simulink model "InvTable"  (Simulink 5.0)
settings: Solver=FixedStepDiscrete  StartTime=0.0  StopTime=inf  FixedStep=samplePeriod  RelTol=1e-3
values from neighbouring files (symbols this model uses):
  a0 = zeros(1, nAct)    [initialize.m]    (also in quake.m = 0; rspect.m = 1)
  azMask = zeros(nAcc, 1)    [initialize.m]
  bal = [[ 1  1  1  1  0  0  0  0  0  0  0  0]    [initialize.m]
  cmap = jet    [initialize.m]    (also in tableAnimation.m = self.cmap)
  ea_t = zeros(3, nAcc)    [initialize.m]
  faces = nAct               			+ [ 1  2  3  4    [initialize.m]    (also in tableAnimation.m = self.faces)
  flowCanon = 63090.2    [initialize.m]
  fmax = zeros(nAct, 1)    [initialize.m]
  gasConstant = 1.8    [initialize.m]
  gee = 1.0    (= 1)    [initialize.m]    (also in accelA2T.m = h(24); accelT2A.m = h(24); Test.m)
  iactParamsX = [actParamsX, dfGain, solver]    [initialize.m]
  iactParamsY = [actParamsY, dfGain, solver]    [initialize.m]
  iactParamsZ = [actParamsZ, dfGain, solver]    [initialize.m]
  inertia = [Ixx 0 0; 0 Iyy 0; 0 0 Izz]    [initialize.m]
  inertiaCanon = 0.1130    (= 0.113)    [initialize.m]
  linAccelCanon = 9800.0    (= 9800)    [initialize.m]    (also in accelA2T.m = h(19); accelT2A.m = h(19); Test.m)
  lines = nAct               			+ [ 1  2  3  4  1    				5  6  7  8  5    				9 10 11 12  9    				0  2  6 10       				0  3  7 11       				0  4  8 12  0];  	lines(find(lines==nAct)) = 0    [initialize.m]    (also in tableAnimation.m = self.lines; viewer.m = 1)
  linVelocCanon = 1000.0    (= 1000)    [initialize.m]    (also in Test.m)
  mass = [massX massY massZ]'    [initialize.m]
  massCanon = 0.4535924e-06    (= 4.535924e-07)    [initialize.m]
  maxDispl = [maxDisplX  			maxDisplY  			maxDisplZ  			maxDisplZ * linVelocCanon / rollRadius  * 180/pi  			maxDisplZ * linVelocCanon / pitchRadius * 180/pi  			min(maxDisplX, maxDisplY) * linVelocCanon / yawRadius * 180/pi]    [initialize.m]
  maxOilVolume = volume * (1 - (precharge/supplyPress)^(1/gasConstant))    (= 32.2704137442)    [initialize.m]
  maxVeloc = [maxVelocX  			maxVelocY  			maxVelocZ  			maxVelocZ * linVelocCanon / rollRadius  * 180/pi  			maxVelocZ * linVelocCanon / pitchRadius * 180/pi  			min(maxVelocX, maxVelocY) * linVelocCanon / yawRadius * 180/pi]    [initialize.m]
  minDispl = -maxDispl    [initialize.m]
  minVeloc = -maxVeloc    [initialize.m]
  nAct = size(rt_t, 2)    [initialize.m]    (also in tableAnimation.m = self.nAct)
  precharge = 2000    [initialize.m]
  pumpFlow = 1e10    (= 10000000000)    [initialize.m]
  ra_t = [  -20.0   -20.0   -92.0 -2590.0  2590.0   -62.0 -2133.0 -2133.0  2133.0  2133.0   -62.0    [initialize.m]    (also in accelA2T.m = [-h9   -h9 -h15 -h10  h10 -h14 -h12 -h12  h12  h12 -h16; accelT2A.m = [-h9   -h9 -h15 -h10  h10 -h14 -h12 -h12  h12  h12 -h16)
  rb_w = [-5692.1 -5692.1  5692.1  5692.1 -2500.0 -2500.0  2500.0  2500.0 -2400.0 -2400.0  2400.0  2400.0    [initialize.m]    (also in tableAnimation.m = rtxrb_w(:,end-nAct+1:end); positT2A.m = [-h4 -h4  h4  h4 -h1 -h1  h1  h1 -h6 -h6  h6  h6)
  returnPress = 50    [initialize.m]
  rgt = -rtg    [initialize.m]
  roll = tbl(4)    [positT2A.m]
  rotAccelCanon = 1    [initialize.m]    (also in accelA2T.m = h(22); accelT2A.m = h(22); Test.m)
  rotForceCanon = 1000    [initialize.m]    (also in forceA2T.m = h(23); Test.m)
  rotVelocCanon = 1    [initialize.m]    (also in accelA2T.m = h(21); accelT2A.m = h(21); Test.m)
  rt_t = [-3106.4 -3106.4  3106.4  3106.4 -2500.0 -2500.0  2500.0  2500.0 -2400.0 -2400.0  2400.0  2400.0    [initialize.m]    (also in positT2A.m = [rt_tx rt_ty rt_tz])
  rtg = cg    [initialize.m]
  rtx_t = [rt_t	topPlane.topLeft(:)  topPlane.topRight(:)  					topPlane.botRight(:) topPlane.botLeft(:)   					midPlane.topLeft(:)  midPlane.topRight(:)  					midPlane.botRight(:) midPlane.botLeft(:)   					botPlane.topLeft(:)  botPlane.topRight(:)  					botPlane.botRight(:) botPlane.botLeft(:)]    [initialize.m]
  samplePeriod = 1/1024    (= 0.0009765625)    [initialize.m]    (also in viewer.m = eval(getHeaderValue(header, 'DELTA_T')))
  supplyPress = 3000    [initialize.m]
  volume = 160    [initialize.m]    (also in quake.m = volume / 231.0)
  volumeCanon = 3785412.0    (= 3785412)    [initialize.m]
  zlim = [min(rb_w(3,:)) 2*halfLengthZ*lengthCanon]    [initialize.m]
undefined symbols (not defined in the file or in its folder): magnitude
libraries: aerospace x51, simulink x26, simulink_extras x1
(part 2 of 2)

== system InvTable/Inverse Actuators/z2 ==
  note: Parameter vector: 1: oil bulk modulus (force/displ^2) 2: servovalve natural frequency (Hz) 3: servovalve damping ratio 4: servovalve overlap 5: rated pressure (force/displ^2) 6: flow at rated pressure (displ^3/sec) 7: actuator piston area 1 (displ^2) 8: actuator piston area 2 (displ^2) 9: actuator usable stroke 1 (displ) 10: actuator usable stroke 2 (displ) 11: actuator end cushion length 1 (displ) 12: actuator end cushion length 2 (displ) 13: actuator parasitic damping factor 14: cross-chamber leakage factor (flow/press) 15: ratio port openings according to area 16: sample period (sec) Conversion factors used for converting signals from external (user) to internal (canonical) units: 17: displacement 18: velocity 19: force 20: pressure 21: flow Other: 22: delta-F feedback gain 23: inverse solver (0: exact, 1: approx)
  note: Note: "1" and "2" denote actuator cylinders on either side of the actuator piston. With positive valve drive, oil is ported into cylinder 1, resulting in positive displacement.
  note: Auxiliary diagnostic output vector: 1: valve opening 2: C1 pressure 3: C2 pressure 4: delta pressure 5: force 6: velocity 7: C1 flow 8: C2 flow 9: total flow 10: kinematic flow 11: compressibility flow 12: leakage flow 13: iteration error
  displ : Inport
  veloc : Inport  Port=2
  force : Inport  Port=3
  spl press : Inport  Port=4
  rtn press : Inport  Port=5
  abs : Abs
  invactuator : S-Function  FunctionName=invactuator  Parameters=params
  total flow sel : Selector  Elements=9  InputPortWidth=13
  cmd : Outport
  flow : Outport  Port=2
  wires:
  abs/1 -> flow/1
  total flow sel/1 -> abs/1
  invactuator/2 -> total flow sel/1
  force/1 -> invactuator/3
  veloc/1 -> invactuator/2
  invactuator/1 -> cmd/1
  displ/1 -> invactuator/1
  rtn press/1 -> invactuator/5
  spl press/1 -> invactuator/4

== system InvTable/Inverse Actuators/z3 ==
  note: Auxiliary diagnostic output vector: 1: valve opening 2: C1 pressure 3: C2 pressure 4: delta pressure 5: force 6: velocity 7: C1 flow 8: C2 flow 9: total flow 10: kinematic flow 11: compressibility flow 12: leakage flow 13: iteration error
  note: Note: "1" and "2" denote actuator cylinders on either side of the actuator piston. With positive valve drive, oil is ported into cylinder 1, resulting in positive displacement.
  note: Parameter vector: 1: oil bulk modulus (force/displ^2) 2: servovalve natural frequency (Hz) 3: servovalve damping ratio 4: servovalve overlap 5: rated pressure (force/displ^2) 6: flow at rated pressure (displ^3/sec) 7: actuator piston area 1 (displ^2) 8: actuator piston area 2 (displ^2) 9: actuator usable stroke 1 (displ) 10: actuator usable stroke 2 (displ) 11: actuator end cushion length 1 (displ) 12: actuator end cushion length 2 (displ) 13: actuator parasitic damping factor 14: cross-chamber leakage factor (flow/press) 15: ratio port openings according to area 16: sample period (sec) Conversion factors used for converting signals from external (user) to internal (canonical) units: 17: displacement 18: velocity 19: force 20: pressure 21: flow Other: 22: delta-F feedback gain 23: inverse solver (0: exact, 1: approx)
  displ : Inport
  veloc : Inport  Port=2
  force : Inport  Port=3
  spl press : Inport  Port=4
  rtn press : Inport  Port=5
  abs : Abs
  invactuator : S-Function  FunctionName=invactuator  Parameters=params
  total flow sel : Selector  Elements=9  InputPortWidth=13
  cmd : Outport
  flow : Outport  Port=2
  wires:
  spl press/1 -> invactuator/4
  rtn press/1 -> invactuator/5
  displ/1 -> invactuator/1
  invactuator/1 -> cmd/1
  veloc/1 -> invactuator/2
  force/1 -> invactuator/3
  invactuator/2 -> total flow sel/1
  total flow sel/1 -> abs/1
  abs/1 -> flow/1

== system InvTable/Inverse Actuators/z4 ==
  note: Parameter vector: 1: oil bulk modulus (force/displ^2) 2: servovalve natural frequency (Hz) 3: servovalve damping ratio 4: servovalve overlap 5: rated pressure (force/displ^2) 6: flow at rated pressure (displ^3/sec) 7: actuator piston area 1 (displ^2) 8: actuator piston area 2 (displ^2) 9: actuator usable stroke 1 (displ) 10: actuator usable stroke 2 (displ) 11: actuator end cushion length 1 (displ) 12: actuator end cushion length 2 (displ) 13: actuator parasitic damping factor 14: cross-chamber leakage factor (flow/press) 15: ratio port openings according to area 16: sample period (sec) Conversion factors used for converting signals from external (user) to internal (canonical) units: 17: displacement 18: velocity 19: force 20: pressure 21: flow Other: 22: delta-F feedback gain 23: inverse solver (0: exact, 1: approx)
  note: Note: "1" and "2" denote actuator cylinders on either side of the actuator piston. With positive valve drive, oil is ported into cylinder 1, resulting in positive displacement.
  note: Auxiliary diagnostic output vector: 1: valve opening 2: C1 pressure 3: C2 pressure 4: delta pressure 5: force 6: velocity 7: C1 flow 8: C2 flow 9: total flow 10: kinematic flow 11: compressibility flow 12: leakage flow 13: iteration error
  displ : Inport
  veloc : Inport  Port=2
  force : Inport  Port=3
  spl press : Inport  Port=4
  rtn press : Inport  Port=5
  abs : Abs
  invactuator : S-Function  FunctionName=invactuator  Parameters=params
  total flow sel : Selector  Elements=9  InputPortWidth=13
  cmd : Outport
  flow : Outport  Port=2
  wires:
  abs/1 -> flow/1
  total flow sel/1 -> abs/1
  invactuator/2 -> total flow sel/1
  force/1 -> invactuator/3
  veloc/1 -> invactuator/2
  invactuator/1 -> cmd/1
  displ/1 -> invactuator/1
  rtn press/1 -> invactuator/5
  spl press/1 -> invactuator/4

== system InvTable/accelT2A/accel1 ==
  linacc : Inport
  rotacc : Inport  Port=2
  rotvel : Inport  Port=3
  Sum : Sum  Inputs=+++
  crossprod1 : aerospace/Axes Transformations/3x3 cross product
  crossprod2 : aerospace/Axes Transformations/3x3 cross product
  crossprod3 : aerospace/Axes Transformations/3x3 cross product
  dotprod : simulink/Math Operations/Dot Product
  orient : Constant  Value=ea_t(:,id)
  ra_t : Constant  Value=ra_t(:,id)
  out : Outport
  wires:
  crossprod2/1 -> crossprod3/2
  crossprod3/1 -> Sum/3
  rotvel/1 -> crossprod3/1, crossprod2/1
  crossprod1/1 -> Sum/2
  ra_t/1 -> crossprod2/2, crossprod1/2
  rotacc/1 -> crossprod1/1
  Sum/1 -> dotprod/1
  linacc/1 -> Sum/1
  dotprod/1 -> out/1
  orient/1 -> dotprod/2

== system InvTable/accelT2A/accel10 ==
  linacc : Inport
  rotacc : Inport  Port=2
  rotvel : Inport  Port=3
  Sum : Sum  Inputs=+++
  crossprod1 : aerospace/Axes Transformations/3x3 cross product
  crossprod2 : aerospace/Axes Transformations/3x3 cross product
  crossprod3 : aerospace/Axes Transformations/3x3 cross product
  dotprod : simulink/Math Operations/Dot Product
  orient : Constant  Value=ea_t(:,id)
  ra_t : Constant  Value=ra_t(:,id)
  out : Outport
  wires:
  orient/1 -> dotprod/2
  dotprod/1 -> out/1
  linacc/1 -> Sum/1
  Sum/1 -> dotprod/1
  rotacc/1 -> crossprod1/1
  ra_t/1 -> crossprod1/2, crossprod2/2
  crossprod1/1 -> Sum/2
  rotvel/1 -> crossprod2/1, crossprod3/1
  crossprod3/1 -> Sum/3
  crossprod2/1 -> crossprod3/2

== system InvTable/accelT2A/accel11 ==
  linacc : Inport
  rotacc : Inport  Port=2
  rotvel : Inport  Port=3
  Sum : Sum  Inputs=+++
  crossprod1 : aerospace/Axes Transformations/3x3 cross product
  crossprod2 : aerospace/Axes Transformations/3x3 cross product
  crossprod3 : aerospace/Axes Transformations/3x3 cross product
  dotprod : simulink/Math Operations/Dot Product
  orient : Constant  Value=ea_t(:,id)
  ra_t : Constant  Value=ra_t(:,id)
  out : Outport
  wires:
  crossprod2/1 -> crossprod3/2
  crossprod3/1 -> Sum/3
  rotvel/1 -> crossprod3/1, crossprod2/1
  crossprod1/1 -> Sum/2
  ra_t/1 -> crossprod2/2, crossprod1/2
  rotacc/1 -> crossprod1/1
  Sum/1 -> dotprod/1
  linacc/1 -> Sum/1
  dotprod/1 -> out/1
  orient/1 -> dotprod/2

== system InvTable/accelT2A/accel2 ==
  linacc : Inport
  rotacc : Inport  Port=2
  rotvel : Inport  Port=3
  Sum : Sum  Inputs=+++
  crossprod1 : aerospace/Axes Transformations/3x3 cross product
  crossprod2 : aerospace/Axes Transformations/3x3 cross product
  crossprod3 : aerospace/Axes Transformations/3x3 cross product
  dotprod : simulink/Math Operations/Dot Product
  orient : Constant  Value=ea_t(:,id)
  ra_t : Constant  Value=ra_t(:,id)
  out : Outport
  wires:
  orient/1 -> dotprod/2
  dotprod/1 -> out/1
  linacc/1 -> Sum/1
  Sum/1 -> dotprod/1
  rotacc/1 -> crossprod1/1
  ra_t/1 -> crossprod1/2, crossprod2/2
  crossprod1/1 -> Sum/2
  rotvel/1 -> crossprod2/1, crossprod3/1
  crossprod3/1 -> Sum/3
  crossprod2/1 -> crossprod3/2

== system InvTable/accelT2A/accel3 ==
  linacc : Inport
  rotacc : Inport  Port=2
  rotvel : Inport  Port=3
  Sum : Sum  Inputs=+++
  crossprod1 : aerospace/Axes Transformations/3x3 cross product
  crossprod2 : aerospace/Axes Transformations/3x3 cross product
  crossprod3 : aerospace/Axes Transformations/3x3 cross product
  dotprod : simulink/Math Operations/Dot Product
  orient : Constant  Value=ea_t(:,id)
  ra_t : Constant  Value=ra_t(:,id)
  out : Outport
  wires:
  crossprod2/1 -> crossprod3/2
  crossprod3/1 -> Sum/3
  rotvel/1 -> crossprod3/1, crossprod2/1
  crossprod1/1 -> Sum/2
  ra_t/1 -> crossprod2/2, crossprod1/2
  rotacc/1 -> crossprod1/1
  Sum/1 -> dotprod/1
  linacc/1 -> Sum/1
  dotprod/1 -> out/1
  orient/1 -> dotprod/2

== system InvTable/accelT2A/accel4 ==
  linacc : Inport
  rotacc : Inport  Port=2
  rotvel : Inport  Port=3
  Sum : Sum  Inputs=+++
  crossprod1 : aerospace/Axes Transformations/3x3 cross product
  crossprod2 : aerospace/Axes Transformations/3x3 cross product
  crossprod3 : aerospace/Axes Transformations/3x3 cross product
  dotprod : simulink/Math Operations/Dot Product
  orient : Constant  Value=ea_t(:,id)
  ra_t : Constant  Value=ra_t(:,id)
  out : Outport
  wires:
  orient/1 -> dotprod/2
  dotprod/1 -> out/1
  linacc/1 -> Sum/1
  Sum/1 -> dotprod/1
  rotacc/1 -> crossprod1/1
  ra_t/1 -> crossprod1/2, crossprod2/2
  crossprod1/1 -> Sum/2
  rotvel/1 -> crossprod2/1, crossprod3/1
  crossprod3/1 -> Sum/3
  crossprod2/1 -> crossprod3/2

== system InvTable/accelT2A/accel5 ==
  linacc : Inport
  rotacc : Inport  Port=2
  rotvel : Inport  Port=3
  Sum : Sum  Inputs=+++
  crossprod1 : aerospace/Axes Transformations/3x3 cross product
  crossprod2 : aerospace/Axes Transformations/3x3 cross product
  crossprod3 : aerospace/Axes Transformations/3x3 cross product
  dotprod : simulink/Math Operations/Dot Product
  orient : Constant  Value=ea_t(:,id)
  ra_t : Constant  Value=ra_t(:,id)
  out : Outport
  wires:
  crossprod2/1 -> crossprod3/2
  crossprod3/1 -> Sum/3
  rotvel/1 -> crossprod3/1, crossprod2/1
  crossprod1/1 -> Sum/2
  ra_t/1 -> crossprod2/2, crossprod1/2
  rotacc/1 -> crossprod1/1
  Sum/1 -> dotprod/1
  linacc/1 -> Sum/1
  dotprod/1 -> out/1
  orient/1 -> dotprod/2

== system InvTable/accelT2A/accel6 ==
  linacc : Inport
  rotacc : Inport  Port=2
  rotvel : Inport  Port=3
  Sum : Sum  Inputs=+++
  crossprod1 : aerospace/Axes Transformations/3x3 cross product
  crossprod2 : aerospace/Axes Transformations/3x3 cross product
  crossprod3 : aerospace/Axes Transformations/3x3 cross product
  dotprod : simulink/Math Operations/Dot Product
  orient : Constant  Value=ea_t(:,id)
  ra_t : Constant  Value=ra_t(:,id)
  out : Outport
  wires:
  orient/1 -> dotprod/2
  dotprod/1 -> out/1
  linacc/1 -> Sum/1
  Sum/1 -> dotprod/1
  rotacc/1 -> crossprod1/1
  ra_t/1 -> crossprod1/2, crossprod2/2
  crossprod1/1 -> Sum/2
  rotvel/1 -> crossprod2/1, crossprod3/1
  crossprod3/1 -> Sum/3
  crossprod2/1 -> crossprod3/2

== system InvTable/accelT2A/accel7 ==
  linacc : Inport
  rotacc : Inport  Port=2
  rotvel : Inport  Port=3
  Sum : Sum  Inputs=+++
  crossprod1 : aerospace/Axes Transformations/3x3 cross product
  crossprod2 : aerospace/Axes Transformations/3x3 cross product
  crossprod3 : aerospace/Axes Transformations/3x3 cross product
  dotprod : simulink/Math Operations/Dot Product
  orient : Constant  Value=ea_t(:,id)
  ra_t : Constant  Value=ra_t(:,id)
  out : Outport
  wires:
  crossprod2/1 -> crossprod3/2
  crossprod3/1 -> Sum/3
  rotvel/1 -> crossprod3/1, crossprod2/1
  crossprod1/1 -> Sum/2
  ra_t/1 -> crossprod2/2, crossprod1/2
  rotacc/1 -> crossprod1/1
  Sum/1 -> dotprod/1
  linacc/1 -> Sum/1
  dotprod/1 -> out/1
  orient/1 -> dotprod/2

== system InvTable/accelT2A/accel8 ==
  linacc : Inport
  rotacc : Inport  Port=2
  rotvel : Inport  Port=3
  Sum : Sum  Inputs=+++
  crossprod1 : aerospace/Axes Transformations/3x3 cross product
  crossprod2 : aerospace/Axes Transformations/3x3 cross product
  crossprod3 : aerospace/Axes Transformations/3x3 cross product
  dotprod : simulink/Math Operations/Dot Product
  orient : Constant  Value=ea_t(:,id)
  ra_t : Constant  Value=ra_t(:,id)
  out : Outport
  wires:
  orient/1 -> dotprod/2
  dotprod/1 -> out/1
  linacc/1 -> Sum/1
  Sum/1 -> dotprod/1
  rotacc/1 -> crossprod1/1
  ra_t/1 -> crossprod1/2, crossprod2/2
  crossprod1/1 -> Sum/2
  rotvel/1 -> crossprod2/1, crossprod3/1
  crossprod3/1 -> Sum/3
  crossprod2/1 -> crossprod3/2

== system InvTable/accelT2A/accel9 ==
  linacc : Inport
  rotacc : Inport  Port=2
  rotvel : Inport  Port=3
  Sum : Sum  Inputs=+++
  crossprod1 : aerospace/Axes Transformations/3x3 cross product
  crossprod2 : aerospace/Axes Transformations/3x3 cross product
  crossprod3 : aerospace/Axes Transformations/3x3 cross product
  dotprod : simulink/Math Operations/Dot Product
  orient : Constant  Value=ea_t(:,id)
  ra_t : Constant  Value=ra_t(:,id)
  out : Outport
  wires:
  crossprod2/1 -> crossprod3/2
  crossprod3/1 -> Sum/3
  rotvel/1 -> crossprod3/1, crossprod2/1
  crossprod1/1 -> Sum/2
  ra_t/1 -> crossprod2/2, crossprod1/2
  rotacc/1 -> crossprod1/1
  Sum/1 -> dotprod/1
  linacc/1 -> Sum/1
  dotprod/1 -> out/1
  orient/1 -> dotprod/2

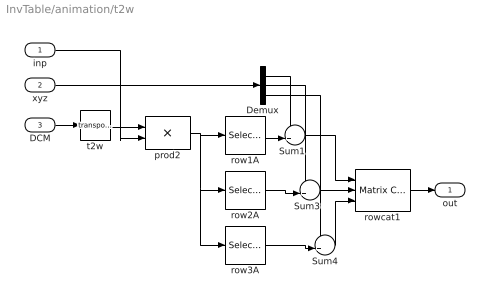
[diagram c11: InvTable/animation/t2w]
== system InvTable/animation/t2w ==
  inp : Inport
  xyz : Inport  Port=2
  DCM : Inport  Port=3
  Demux : Demux  Outputs=3
  Sum1 : Sum  Inputs=++|
  Sum3 : Sum  Inputs=++|
  Sum4 : Sum  Inputs=++|
  prod2 : Product  Multiplication=Matrix(*)
  row1A : Selector  InputType=Matrix  Elements=[1 3]  Columns=-1  InputPortWidth=3
  row2A : Selector  InputType=Matrix  Elements=[1 3]  Rows=2  Columns=-1  InputPortWidth=3
  row3A : Selector  InputType=Matrix  Elements=[1 3]  Rows=3  Columns=-1  InputPortWidth=3
  rowcat1 : simulink/Math Operations/Matrix Concatenation  numInports=3  catMethod=Vertical
  t2w : Math  Operator=transpose
  out : Outport
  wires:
  t2w/1 -> prod2/1
  Sum4/1 -> rowcat1/3
  Sum1/1 -> rowcat1/1
  Sum3/1 -> rowcat1/2
  Demux/3 -> Sum4/1
  Demux/2 -> Sum3/1
  row3A/1 -> Sum4/2
  row2A/1 -> Sum3/2
  Demux/1 -> Sum1/1
  prod2/1 -> row2A/1, row3A/1, row1A/1
  DCM/1 -> t2w/1
  inp/1 -> prod2/2
  rowcat1/1 -> out/1
  row1A/1 -> Sum1/2
  xyz/1 -> Demux/1

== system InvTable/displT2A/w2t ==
  inp : Inport
  xyz : Inport  Port=2
  DCM : Inport  Port=3
  Demux : Demux  Outputs=3
  Sum5 : Sum  Inputs=-+|
  Sum6 : Sum  Inputs=-+|
  Sum7 : Sum  Inputs=-+|
  prod : Product  Multiplication=Matrix(*)
  row1A : Selector  InputType=Matrix  Elements=[1 3]  Columns=-1  InputPortWidth=3
  row2A : Selector  InputType=Matrix  Elements=[1 3]  Rows=2  Columns=-1  InputPortWidth=3
  row3A : Selector  InputType=Matrix  Elements=[1 3]  Rows=3  Columns=-1  InputPortWidth=3
  rowcat : simulink/Math Operations/Matrix Concatenation  numInports=3  catMethod=Vertical
  out : Outport
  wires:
  DCM/1 -> prod/1
  prod/1 -> out/1
  rowcat/1 -> prod/2
  inp/1 -> row3A/1, row2A/1, row1A/1
  xyz/1 -> Demux/1
  row1A/1 -> Sum5/2
  Demux/1 -> Sum5/1
  row2A/1 -> Sum6/2
  row3A/1 -> Sum7/2
  Demux/2 -> Sum6/1
  Demux/3 -> Sum7/1
  Sum6/1 -> rowcat/2
  Sum5/1 -> rowcat/1
  Sum7/1 -> rowcat/3

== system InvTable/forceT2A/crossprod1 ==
  A : Inport
  B : Inport  Port=2
  colA : Selector  InputType=Matrix  Elements=[1 3]  Rows=-1  Columns=id  InputPortWidth=3
  colB : Selector  InputType=Matrix  Elements=[1 3]  Rows=-1  Columns=id  InputPortWidth=3
  crossprod : aerospace/Axes Transformations/3x3 cross product
  AxB : Outport
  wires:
  crossprod/1 -> AxB/1
  B/1 -> colB/1
  A/1 -> colA/1
  colB/1 -> crossprod/2
  colA/1 -> crossprod/1

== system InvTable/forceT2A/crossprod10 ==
  A : Inport
  B : Inport  Port=2
  colA : Selector  InputType=Matrix  Elements=[1 3]  Rows=-1  Columns=id  InputPortWidth=3
  colB : Selector  InputType=Matrix  Elements=[1 3]  Rows=-1  Columns=id  InputPortWidth=3
  crossprod : aerospace/Axes Transformations/3x3 cross product
  AxB : Outport
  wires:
  colA/1 -> crossprod/1
  colB/1 -> crossprod/2
  A/1 -> colA/1
  B/1 -> colB/1
  crossprod/1 -> AxB/1

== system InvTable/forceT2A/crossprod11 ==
  A : Inport
  B : Inport  Port=2
  colA : Selector  InputType=Matrix  Elements=[1 3]  Rows=-1  Columns=id  InputPortWidth=3
  colB : Selector  InputType=Matrix  Elements=[1 3]  Rows=-1  Columns=id  InputPortWidth=3
  crossprod : aerospace/Axes Transformations/3x3 cross product
  AxB : Outport
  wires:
  crossprod/1 -> AxB/1
  B/1 -> colB/1
  A/1 -> colA/1
  colB/1 -> crossprod/2
  colA/1 -> crossprod/1

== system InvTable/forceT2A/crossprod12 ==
  A : Inport
  B : Inport  Port=2
  colA : Selector  InputType=Matrix  Elements=[1 3]  Rows=-1  Columns=id  InputPortWidth=3
  colB : Selector  InputType=Matrix  Elements=[1 3]  Rows=-1  Columns=id  InputPortWidth=3
  crossprod : aerospace/Axes Transformations/3x3 cross product
  AxB : Outport
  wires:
  colA/1 -> crossprod/1
  colB/1 -> crossprod/2
  A/1 -> colA/1
  B/1 -> colB/1
  crossprod/1 -> AxB/1

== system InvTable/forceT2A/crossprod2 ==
  A : Inport
  B : Inport  Port=2
  colA : Selector  InputType=Matrix  Elements=[1 3]  Rows=-1  Columns=id  InputPortWidth=3
  colB : Selector  InputType=Matrix  Elements=[1 3]  Rows=-1  Columns=id  InputPortWidth=3
  crossprod : aerospace/Axes Transformations/3x3 cross product
  AxB : Outport
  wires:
  colA/1 -> crossprod/1
  colB/1 -> crossprod/2
  A/1 -> colA/1
  B/1 -> colB/1
  crossprod/1 -> AxB/1

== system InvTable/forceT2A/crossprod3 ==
  A : Inport
  B : Inport  Port=2
  colA : Selector  InputType=Matrix  Elements=[1 3]  Rows=-1  Columns=id  InputPortWidth=3
  colB : Selector  InputType=Matrix  Elements=[1 3]  Rows=-1  Columns=id  InputPortWidth=3
  crossprod : aerospace/Axes Transformations/3x3 cross product
  AxB : Outport
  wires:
  crossprod/1 -> AxB/1
  B/1 -> colB/1
  A/1 -> colA/1
  colB/1 -> crossprod/2
  colA/1 -> crossprod/1

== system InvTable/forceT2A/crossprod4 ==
  A : Inport
  B : Inport  Port=2
  colA : Selector  InputType=Matrix  Elements=[1 3]  Rows=-1  Columns=id  InputPortWidth=3
  colB : Selector  InputType=Matrix  Elements=[1 3]  Rows=-1  Columns=id  InputPortWidth=3
  crossprod : aerospace/Axes Transformations/3x3 cross product
  AxB : Outport
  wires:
  colA/1 -> crossprod/1
  colB/1 -> crossprod/2
  A/1 -> colA/1
  B/1 -> colB/1
  crossprod/1 -> AxB/1

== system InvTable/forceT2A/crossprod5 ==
  A : Inport
  B : Inport  Port=2
  colA : Selector  InputType=Matrix  Elements=[1 3]  Rows=-1  Columns=id  InputPortWidth=3
  colB : Selector  InputType=Matrix  Elements=[1 3]  Rows=-1  Columns=id  InputPortWidth=3
  crossprod : aerospace/Axes Transformations/3x3 cross product
  AxB : Outport
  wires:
  crossprod/1 -> AxB/1
  B/1 -> colB/1
  A/1 -> colA/1
  colB/1 -> crossprod/2
  colA/1 -> crossprod/1

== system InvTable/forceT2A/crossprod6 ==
  A : Inport
  B : Inport  Port=2
  colA : Selector  InputType=Matrix  Elements=[1 3]  Rows=-1  Columns=id  InputPortWidth=3
  colB : Selector  InputType=Matrix  Elements=[1 3]  Rows=-1  Columns=id  InputPortWidth=3
  crossprod : aerospace/Axes Transformations/3x3 cross product
  AxB : Outport
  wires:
  colA/1 -> crossprod/1
  colB/1 -> crossprod/2
  A/1 -> colA/1
  B/1 -> colB/1
  crossprod/1 -> AxB/1

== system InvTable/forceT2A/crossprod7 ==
  A : Inport
  B : Inport  Port=2
  colA : Selector  InputType=Matrix  Elements=[1 3]  Rows=-1  Columns=id  InputPortWidth=3
  colB : Selector  InputType=Matrix  Elements=[1 3]  Rows=-1  Columns=id  InputPortWidth=3
  crossprod : aerospace/Axes Transformations/3x3 cross product
  AxB : Outport
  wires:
  crossprod/1 -> AxB/1
  B/1 -> colB/1
  A/1 -> colA/1
  colB/1 -> crossprod/2
  colA/1 -> crossprod/1

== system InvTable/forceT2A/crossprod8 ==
  A : Inport
  B : Inport  Port=2
  colA : Selector  InputType=Matrix  Elements=[1 3]  Rows=-1  Columns=id  InputPortWidth=3
  colB : Selector  InputType=Matrix  Elements=[1 3]  Rows=-1  Columns=id  InputPortWidth=3
  crossprod : aerospace/Axes Transformations/3x3 cross product
  AxB : Outport
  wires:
  colA/1 -> crossprod/1
  colB/1 -> crossprod/2
  A/1 -> colA/1
  B/1 -> colB/1
  crossprod/1 -> AxB/1

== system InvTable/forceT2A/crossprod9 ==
  A : Inport
  B : Inport  Port=2
  colA : Selector  InputType=Matrix  Elements=[1 3]  Rows=-1  Columns=id  InputPortWidth=3
  colB : Selector  InputType=Matrix  Elements=[1 3]  Rows=-1  Columns=id  InputPortWidth=3
  crossprod : aerospace/Axes Transformations/3x3 cross product
  AxB : Outport
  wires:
  crossprod/1 -> AxB/1
  B/1 -> colB/1
  A/1 -> colA/1
  colB/1 -> crossprod/2
  colA/1 -> crossprod/1
